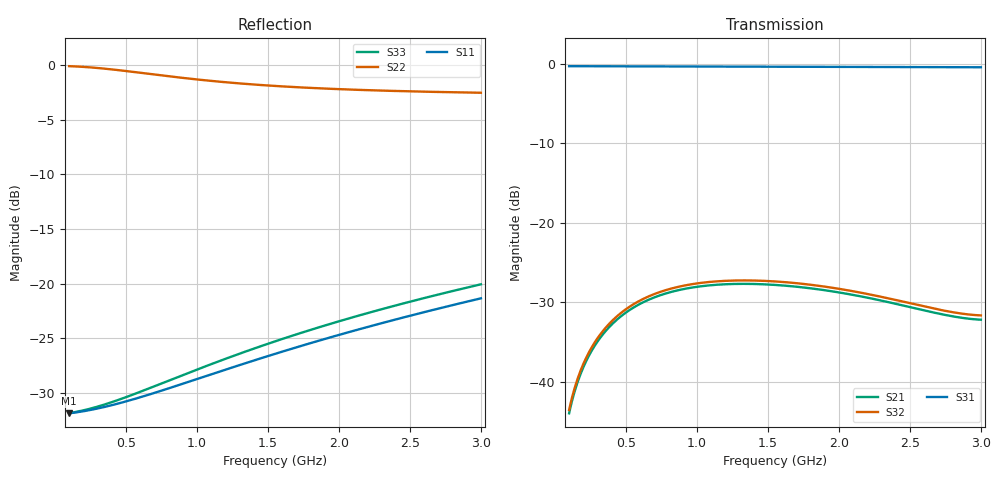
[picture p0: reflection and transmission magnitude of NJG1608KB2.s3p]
!  Port1:P1, Port2:P2, Port3:PC
# hz S ri R 50
! 3 Port Network Data from SP1.SP block
! freq  reS11  imS11  reS12  imS12  reS13  imS13
!  reS21  imS21
!  reS22  imS22  reS23  imS23
!  reS31  imS31  reS32  imS32
!  reS33  imS33
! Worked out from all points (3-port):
!   291 points, 100 MHz to 3 GHz, reference 50 ohm
!   strongest paths, dB at 100 MHz, 820 MHz, 1.55 GHz, 2.28 GHz, 3 GHz:
!     S31: -0.3, -0.3, -0.3, -0.4, -0.4
!     S32: -43.6, -28.3, -27.4, -29.3, -31.7
!     S21: -44.0, -28.7, -27.8, -29.7, -32.2
!   lowest |S11| = -31.9 dB at 100 MHz (marker M1), VSWR 1.05, Z = 52.6 - j0.416 ohm
!   |S11| at or under -10 dB: start of sweep to end of sweep
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1e8  0.0252 -0.00396  0.00173 0.00607  0.969 -0.0232
     0.00173 0.00607  0.9648 -0.2146  0.00179 0.00637
     0.969 -0.0232  0.00179 0.00637  0.0252 -0.00419
1.9e8  0.025 -0.00726  0.00365 0.0111  0.9679 -0.0437
       0.00365 0.0111  0.8995 -0.394  0.00376 0.0117
       0.9679 -0.0437  0.00376 0.0117  0.0251 -0.00771
3.1e8  0.0243 -0.0116  0.00765 0.0167  0.9657 -0.0711
       0.00765 0.0167  0.7625 -0.5971  0.00785 0.0176
       0.9657 -0.0711  0.00785 0.0176  0.0245 -0.0124
4.9e8  0.0226 -0.0179  0.0153 0.022  0.9608 -0.1118
       0.0153 0.022  0.4935 -0.8012  0.0157 0.0233
       0.9608 -0.1118  0.0157 0.0233  0.0232 -0.0191
6.7e8  0.0202 -0.0238  0.0231 0.0237  0.9542 -0.152
       0.0231 0.0237  0.2084 -0.8863  0.0237 0.0254
       0.9542 -0.152  0.0237 0.0254  0.0214 -0.0256
8.6e8  0.0171 -0.0296  0.0299 0.0226  0.9455 -0.1939
       0.0299 0.0226  -0.0625 -0.8774  0.0307 0.0246
       0.9455 -0.1939  0.0307 0.0246  0.019 -0.032
1.09e9  0.0127 -0.0361  0.0355 0.0192  0.9326 -0.2438
        0.0355 0.0192  -0.3227 -0.7839  0.0366 0.0215
        0.9326 -0.2438  0.0366 0.0215  0.0158 -0.0395
1.55e9  0.0018 -0.0477  0.039 0.0112  0.8992 -0.3412
        0.039 0.0112  -0.6337 -0.4924  0.0404 0.0138
        0.8992 -0.3412  0.0404 0.0138  0.00784 -0.0539
2.18e9  -0.0178 -0.0602  0.0336 0.0054  0.8369 -0.4681
        0.0336 0.0054  -0.7634 -0.0885  0.035 0.00816
        0.8369 -0.4681  0.035 0.00816  -0.0067 -0.0724
3e9  -0.0515 -0.0685  0.0212 0.0123  0.727 -0.6179
     0.0212 0.0123  -0.6747 0.3208  0.0213 0.0151
     0.727 -0.6179  0.0213 0.0151  -0.0335 -0.0935
